[IBIS ver]   4.1
[File name]   sprm639a.ibs
[File Rev]   1.0
[Notes]
   IO cell model for C2000
[Date]   Nov 21, 2013
[Source]   File originated at Texas Instruments
[Copyright]   (c) 2012, Texas Instruments Inc.
[Component]   f771553xzwt
[Manufacturer] Texas Instruments
[Package]
| Variable   Typ   Min   Max
R_pkg   0.248   0.104   0.421
L_pkg   3.07E-09   9.51E-10   5.41E-09
C_pkg   7.15E-13   3.27E-13   1.18E-12
[Pin] signal_name   model_name   R_pin   L_pin   C_pin
A11   GPIO84   BCF3385DSHYPBFZ   0.319687   4.33705E-09   7.78071E-13
A12   GPIO153   BCF3350CSHYPBFZ   0.298822   4.20847E-09   6.39259E-13
A13   GPIO149   BCF3350CSHYPBFZ   0.342954   4.55481E-09   6.48797E-13
A14   GPIO81   BCF3385DSHYPBFZ   0.33134   4.4902E-09   7.50504E-13
A15   GPIO77   BCF3385DSHYPBFZ   0.337162   4.66581E-09   6.92522E-13
A16   GPIO73   BCF3385DSHYPBFZ   0.375286   4.90719E-09   9.3949E-13
A17   GPIO70   BCF3335DSHYPBFZ   0.421882   5.41022E-09   9.06764E-13
A2   GPIO97   BCF3385DSHYPBFZ   0.346517   3.88805E-09   7.27628E-13
A3   GPIO94   BCF3385DSHYPBFZ   0.327527   4.38519E-09   8.14171E-13
A4   GPIO92   BCF3385DSHYPBFZ   0.367132   4.84058E-09   8.98899E-13
A5   GPIO90   BCF3385DSHYPBFZ   0.309269   4.27709E-09   6.00141E-13
A6   GPIO6   GPIORETV2_NFS   0.308865   4.3618E-09   6.23916E-13
A7   GPIO2   GPIORETV2_NFS   0.295368   4.05632E-09   6.22769E-13
A8   GPIO163   BCF3350CSHYPBFZ   0.285759   3.62759E-09   7.23531E-13
|*A9,A18,B1,E7,E10,E13,F7,F10,F13,G5   VDDSFL   NC   0.146867   1.37666E-09   6.11163E-13*|
|*G6,H5,H6,L14,L15,M1,M5,M6,N14,N15,P9,R9,V19,W8   VDDSFL   NC   0.156081   1.50618E-09   6.11163E-13*|
B10   GPIO157   BCF3350CSHYPBFZ   0.309235   3.83913E-09   6.87623E-13
B11   GPIO85   BCF3385DSHYPBFZ   0.272894   3.41813E-09   7.01392E-13
B12   GPIO154   BCF3350CSHYPBFZ   0.303603   3.86334E-09   8.09406E-13
B13   GPIO150   BCF3350CSHYPBFZ   0.319404   4.36169E-09   8.51309E-13
B14   GPIO82   BCF3385DSHYPBFZ   0.287611   3.75595E-09   7.91276E-13
B15   GPIO78   BCF3385DSHYPBFZ   0.303045   3.86525E-09   9.89285E-13
B16   GPIO72   BCF3335DSHYPBFZ   0.320566   4.21723E-09   9.70252E-13
B17   GPIO71   BCF3385DSHYPBFZ   0.365339   4.78832E-09   8.84874E-13
B18   GPIO69   BCF3385DSHYPBFZ   0.377633   4.86821E-09   1.02379E-12
B19   GPIO67   BCF3385DSHYPBFZ   0.35161   3.71783E-09   9.11537E-13
B2   GPIO10   BCF183350CSHYPBFZ   0.304557   3.85412E-09   7.12492E-13
B3   GPIO95   BCF3350CSHYPBFZ   0.320186   4.02158E-09   7.8623E-13
B4   GPIO93   BCF3385DSHYPBFZ   0.320914   4.19498E-09   8.33886E-13
B5   GPIO91   BCF3385DSHYPBFZ   0.315637   4.16133E-09   9.379E-13
B6   GPIO7   GPIORETV2_NFS   0.252616   3.27964E-09   7.68154E-13
B7   GPIO3   GPIORETV2_NFS   0.248561   3.29545E-09   7.95932E-13
B8   GPIO164   BCF3350CSHYPBFZ   0.298994   3.61876E-09   6.752E-13
B9   GPIO160   BCF3350CSHYPBFZ   0.247443   3.09689E-09   5.80944E-13
C1   GPIO11   BCF183350CSHYPBFZ   0.307276   4.07789E-09   6.71632E-13
C10   GPIO158   BCF3350CSHYPBFZ   0.251923   3.02701E-09   6.50017E-13
C11   GPIO86   BCF3385DSHYPBFZ   0.240019   2.99169E-09   8.31328E-13
C12   GPIO155   BCF3350CSHYPBFZ   0.283764   3.59088E-09   7.34615E-13
C13   GPIO151   BCF3350CSHYPBFZ   0.25868   3.23014E-09   7.11853E-13
C14   GPIO83   BCF3385DSHYPBFZ   0.295575   3.78014E-09   7.76833E-13
C15   GPIO79   BCF3385DSHYPBFZ   0.31018   4.22638E-09   7.99064E-13
C16   GPIO76   BCF3385DSHYPBFZ   0.290281   3.78138E-09   1.02012E-12
C17   GPIO74   BCF3385DSHYPBFZ   0.323895   4.29426E-09   1.10069E-12
C18   GPIO68   BCF3385DSHYPBFZ   0.335665   3.64035E-09   1.10713E-12
C19   GPIO43   GPIOUSBV4_NFS_7LM   0.321464   3.65132E-09   7.88734E-13
C2   GPIO12   BCF183350CSHYPBFZ   0.292939   3.97645E-09   7.61513E-13
C3   GPIO96   BCF3385DSHYPBFZ   0.261803   3.07199E-09   8.01544E-13
C4   GPIO167   BCF3350CSHYPBFZ   0.294566   3.73299E-09   8.19332E-13
C5   GPIO165   BCF3350CSHYPBFZ   0.272342   3.43944E-09   6.65144E-13
C6   GPIO88   BCF3385DSHYPBFZ   0.259602   3.22338E-09   6.6121E-13
C7   GPIO4   GPIORETV2_NFS   0.215794   2.71638E-09   6.10609E-13
C8   GPIO0   GPIORETV2_NFS   0.244304   3.06821E-09   6.6699E-13
C9   GPIO161   BCF3350CSHYPBFZ   0.241226   2.87469E-09   7.86601E-13
D1   GPIO13   BCF183350CSHYPBFZ   0.299551   4.19571E-09   6.95654E-13
D10   GPIO159   BCF3350CSHYPBFZ   0.191658   2.18732E-09   7.58875E-13
D11   GPIO87   BCF3385DSHYPBFZ   0.22167   2.69751E-09   7.53613E-13
D12   GPIO156   BCF3350CSHYPBFZ   0.222483   2.73461E-09   8.74454E-13
D13   GPIO152   BCF3350CSHYPBFZ   0.248923   3.14502E-09   8.96352E-13
D14   GPIO148   BCF3350CSHYPBFZ   0.327228   4.26288E-09   9.56502E-13
D15   GPIO80   BCF3385DSHYPBFZ   0.325935   4.3086E-09   9.4736E-13
D16   GPIO75   BCF3385DSHYPBFZ   0.345154   4.59742E-09   9.19875E-13
D17   GPIO147   BCF3350CSHYPBFZ   0.26482   3.40869E-09   1.11582E-12
D18   GPIO146   BCF3350CSHYPBFZ   0.318138   3.82793E-09   1.18493E-12
D19   GPIO42   GPIOUSBV4_NFS_7LM   0.315732   4.00436E-09   7.19589E-13
D2   GPIO14   BCF183350CSHYPBFZ   0.307598   4.03173E-09   6.21597E-13
D3   GPIO15   BCF183350CSHYPBFZ   0.252167   3.22666E-09   7.94736E-13
D4   GPIO168   BCF3350CSHYPBFZ   0.226606   2.66721E-09   8.86402E-13
D5   GPIO166   BCF3350CSHYPBFZ   0.237854   3.0172E-09   7.4741E-13
D6   GPIO89   BCF3385DSHYPBFZ   0.206799   2.47062E-09   8.1398E-13
D7   GPIO5   GPIORETV2_NFS   0.192542   2.15668E-09   8.21398E-13
D8   GPIO1   GPIORETV2_NFS   0.168654   2.0599E-09   6.44669E-13
D9   GPIO162   BCF3350CSHYPBFZ   0.20821   2.27434E-09   5.90519E-13
E1   GPIO16   BCF183350CSHYPBFZ   0.314704   4.17604E-09   5.05103E-13
|*E16,F16   VDDSFL2   NC   0.156792   1.71059E-09   4.40263E-13*|
|*E16,F16   VDDSFL2   NC   0.154282   1.6878E-09   4.40263E-13*|
E17   GPIO145   BCF3350CSHYPBFZ   0.21249   2.55446E-09   9.60886E-13
E18   GPIO47   GPIOUSBV4_NFS_7LM   0.253816   3.03959E-09   6.70576E-13
E19   GPIO46   GPIOUSBV4_NFS_7LM   0.294305   3.60496E-09   6.48949E-13
E2   GPIO17   BCF183350CSHYPBFZ   0.257137   3.29303E-09   7.29543E-13
E3   GPIO18   BCF183350CSHYPBFZ   0.258589   3.34891E-09   5.60313E-13
E4   GPIO19   BCF183350CSHYPBFZ   0.27369   3.55971E-09   6.78789E-13
|*E9,E11,F9,F11,G14,G15,J14,J15,K5,K6,P10,P13,R10,R13   VDD   NC  0.171112   1.72645E-09   4.7223E-13*|
F1   GPIO98   BCF3385DSHYPBFZ   0.314572   4.25419E-09   6.22881E-13
F17   GPIO144   BCF3350BSHYPBFZ   0.237538   2.5957E-09   6.13332E-13
F18   GPIO143   BCF3350BSHYPBFZ   0.321464   4.16724E-09   1.01147E-12
F19   XRSn   BQ0491FS_3X2_7LM   0.286137   2.93417E-09   6.60717E-13
F2   GPIO20   BCF183350CSHYPBFZ   0.235787   3.13823E-09   6.44518E-13
F3   GPIO21   BCF183350CSHYPBFZ   0.244247   3.08261E-09   5.66615E-13
|*F4,G4   VDDSFL1833   NC   0.135167   1.53786E-09   5.04299E-13*|
|*F4,G4   VDDSFL1833   NC   0.126166   1.45446E-09   5.04299E-13*|
G1   GPIO99   BCF3385DSHYPBFZ   0.285592   3.81153E-09   7.64347E-13
G18   GPIO133   BCF3350BSHYPBFZ   0.294888   3.819E-09   7.35036E-13
G19   X1   NC   0.262328   2.90312E-09   7.47045E-13
G2   GPIO8   BCF3350CSHYPBFZ   0.264806   3.67528E-09   7.26003E-13
G3   GPIO9   BCF3350CSHYPBFZ   0.252788   3.25417E-09   6.09259E-13
H1   GPIO100   BCF3385DSHYPBFZ   0.263476   3.65228E-09   5.78824E-13
|*H16,H17   VDDSFL1   NC   0.133588   1.49772E-09   6.04206E-13*|
|*H16,H17   VDDSFL1   NC   0.13331   1.49845E-09   6.04206E-13*|
|*H18,H19   VSS   NC   0.232486   2.61579E-09   7.29732E-13*|
H2   GPIO101   BCF3385DSHYPBFZ   0.249794   3.18204E-09   5.27391E-13
H3   GPIO102   BCF3385DSHYPBFZ   0.226173   2.77789E-09   6.83769E-13
H4   VPP   NC   0.125134   1.44032E-09   3.27051E-13
J1   GPIO103   BCF3385DSHYPBFZ   0.287709   3.95912E-09   5.76491E-13
J16   GPIO63   BCF3385DSHYPBFZ   0.263216   2.95033E-09   8.91047E-13
J17   GPIO62   BCF3385DSHYPBFZ   0.30101   3.6262E-09   7.47986E-13
J18   VREGENZ   IQ0440FS_3X2_7LM   0.260757   3.23788E-09   6.52653E-13
J19   X2   NC   0.249184   3.17546E-09   6.96076E-13
J2   GPIO104   BCF3385DSHYPBFZ   0.223555   2.89779E-09   5.79891E-13
J3   GPIO105   BCF3385DSHYPBFZ   0.261577   3.22449E-09   6.38145E-13
J4   GPIO22   BCF3350CSHYPBFZ   0.211796   2.42294E-09   6.4932E-13
K1   GPIO26   BCF3350CSHYPBFZ   0.285128   3.9065E-09   6.35515E-13
K16   GPIO65   BCF3385DSHYPBFZ   0.174096   1.80345E-09   8.82989E-13
K17   GPIO66   BCF3335DSHYPBFZ   0.229966   2.57395E-09   5.41566E-13
K18   GPIO44   BCF3385DSHYPBFZ   0.271389   3.34545E-09   5.75478E-13
K19   GPIO45   BCF3385DSHYPBFZ   0.290096   4.03352E-09   6.51737E-13
K2   GPIO25   BCF3350CSHYPBFZ   0.234189   3.01207E-09   6.61863E-13
K3   GPIO24   BCF3350CSHYPBFZ   0.199766   2.32311E-09   5.45272E-13
K4   GPIO23   BCF3350CSHYPBFZ   0.142595   1.46053E-09   7.05502E-13
L1   GPIO27   BCF3350CSHYPBFZ   0.29442   3.97471E-09   6.61819E-13
L16   GPIO61   BCF3335DSHYPBFZ   0.133751   1.33372E-09   7.57122E-13
L17   GPIO64   BCF3335DSHYPBFZ   0.209578   2.25357E-09   5.83731E-13
L19   GPIO142   BCF3350BSHYPBFZ   0.306503   3.59516E-09   5.37682E-13
L2   GPIO106   BCF3385DSHYPBFZ   0.277201   3.4199E-09   5.17299E-13
L3   GPIO107   BCF3385DSHYPBFZ   0.220847   2.66337E-09   7.07224E-13
L4   GPIO108   BCF3385DSHYPBFZ   0.195261   2.03861E-09   5.37039E-13
M16   GPIO59   BCF3335DSHYPBFZ   0.134266   1.44911E-09   6.89352E-13
M17   GPIO60   BCF3385DSHYPBFZ   0.219583   2.23847E-09   8.61878E-13
M18   GPIO141   BCF3350BSHYPBFZ   0.287892   3.23826E-09   6.16719E-13
M19   GPIO140   BCF3350BSHYPBFZ   0.307057   3.82104E-09   6.32699E-13
M2   GPIO110   BCF3385DSHYPBFZ   0.283588   3.43407E-09   5.00861E-13
M3   GPIO112   BCF3385DSHYPBFZ   0.255848   2.93253E-09   5.7291E-13
M4   GPIO111   BCF3385DSHYPBFZ   0.179094   2.06636E-09   8.32478E-13
N16   GPIO56   BCF3385DSHYPBFZ   0.140094   1.67717E-09   7.26011E-13
N17   GPIO58   BCF3385DSHYPBFZ   0.239696   2.73931E-09   7.19111E-13
N18   GPIO57   BCF3385DSHYPBFZ   0.252681   3.14084E-09   5.55753E-13
N19   GPIO139   BCF3350BSHYPBFZ   0.32263   4.08555E-09   5.86096E-13
N2   GPIO109   BCF3385DSHYPBFZ   0.293848   3.66524E-09   7.64043E-13
N3   GPIO114   BCF3385DSHYPBFZ   0.273962   3.33937E-09   6.65314E-13
N4   GPIO113   BCF3385DSHYPBFZ   0.213519   2.56277E-09   7.61396E-13
|*P1,P5,R5,V7,W1   VSSA   NC   0.128935   1.30292E-09   9.97767E-13*|
|*P1,P5,R5,V7,W1   VSSA   NC   0.128558   1.41788E-09   9.97767E-13*|
|*P1,P5,R5,V7,W1   VSSA   NC   0.131821   1.42996E-09   9.97767E-13*|
|*P1,P5,R5,V7,W1   VSSA   NC   0.147367   1.47463E-09   9.97767E-13*|
|*P1,P5,R5,V7,W1   VSSA   NC   0.148848   1.45141E-09   9.97767E-13*|
|*P1,P5,R5,V7,W1   VSSA   NC   0.131419   1.3196E-09   9.97767E-13*|
P16   GPIO52   BCF3385DSHYPBFZ   0.24655   3.08807E-09   6.49119E-13
P17   GPIO53   BCF3385DSHYPBFZ   0.207708   2.86996E-09   5.95892E-13
P18   GPIO54   BCF3385DSHYPBFZ   0.263121   3.43701E-09   5.40139E-13
P19   GPIO55   BCF3385DSHYPBFZ   0.313207   4.21928E-09   6.49976E-13
P2   ADCINC1   NC   0.311442   4.01529E-09   6.9028E-13
P3   ADCINC3   NC   0.275666   3.47007E-09   7.11166E-13
P4   ADCINC5   NC   0.270084   3.25121E-09   9.143E-13
|*P6,R6   VDDA   NC   0.140595   1.46957E-09   4.04901E-13*|
|*P6,R6   VDDA   NC   0.143704   1.4855E-09   4.04901E-13*|
|*P6,R6   VDDA   NC   0.149119   1.6026E-09   4.04901E-13*|
|*P6,R6   VDDA   NC   0.14411   1.59172E-09   4.04901E-13*|
R1   VREFHI3   NC   0.292156   3.6476E-09   4.74414E-13
|*R11,R12   VDD3VFL   NC   0.117117   1.18661E-09   4.79636E-13*|
|*R11,R12   VDD3VFL   NC   0.115756   1.18172E-09   4.79636E-13*|
R16   GPIO48   BCF3385DSHYPBFZ   0.202473   2.42772E-09   6.9922E-13
R17   GPIO49   BCF3385DSHYPBFZ   0.211152   2.81544E-09   6.94346E-13
R18   GPIO50   BCF3385DSHYPBFZ   0.290055   3.84404E-09   6.44835E-13
R19   GPIO51   BCF3385DSHYPBFZ   0.313144   4.71586E-09   6.56413E-13
R2   ADCINC0   NC   0.318008   3.66132E-09   8.46127E-13
R3   ADCINC2   NC   0.279974   3.28028E-09   9.46719E-13
R4   ADCINC4   NC   0.305712   3.6984E-09   1.01504E-12
T1   ADCINA1   NC   0.379067   4.60718E-09   1.02321E-12
T10   GPIO129   BCF3350BSHYPBFZ   0.168143   2.075E-09   6.72018E-13
T11   GPIO30   BCF3355DSHYPBFZ   0.207085   2.45219E-09   8.10867E-13
T12   GPIO118   BCF3355DSHYPBFZ   0.187417   2.33318E-09   8.67819E-13
T13   GPIO33   BCF3385DSHYPBFZ   0.24449   2.84693E-09   7.57249E-13
T14   GPIO35   BCF3385DSHYPBFZ   0.279565   3.58098E-09   8.13795E-13
T15   GPIO119   BCF3385DSHYPBFZ   0.230666   2.73008E-09   7.94503E-13
T16   GPIO38   BCF3385DSHYPBFZ   0.236446   2.81408E-09   8.58047E-13
T17   GPIO136   BCF3350BSHYPBFZ   0.260209   3.18036E-09   7.40507E-13
T18   GPIO137   BCF3350BSHYPBFZ   0.253664   3.59979E-09   6.57827E-13
T19   GPIO138   BCF3350BSHYPBFZ   0.366548   5.03901E-09   7.07013E-13
T2   ADCINA3   NC   0.327198   4.02466E-09   9.03426E-13
T3   ADCINA5   NC   0.291696   3.43909E-09   8.41751E-13
T4   ADCINCAL0   NC   0.231734   2.60307E-09   7.77891E-13
T5   ADCIND0   NC   0.269236   3.20966E-09   1.0884E-12
T6   ADCIND2   NC   0.236315   2.66335E-09   9.76019E-13
T7   ADCIND4   NC   0.201937   2.21871E-09   8.76865E-13
T8   GPIO122   BCF3350CSHYPBFZ   0.188754   2.03765E-09   7.57926E-13
T9   GPIO125   BCF3350CSHYPBFZ   0.192836   2.24227E-09   5.7875E-13
U1   ADCINA0   NC   0.37235   4.01208E-09   9.42551E-13
U10   GPIO130   BCF3350BSHYPBFZ   0.234168   2.75572E-09   7.21435E-13
U11   GPIO31   BCF3385DSHYPBFZ   0.23223   2.89131E-09   8.5392E-13
U12   GPIO117   BCF3385DSHYPBFZ   0.254774   3.22477E-09   7.05375E-13
U13   GPIO32   BCF3385DSHYPBFZ   0.251017   3.07874E-09   8.00807E-13
U14   GPIO34   BCF3385DSHYPBFZ   0.292993   3.92802E-09   8.95378E-13
U15   GPIO120   BCF3385DSHYPBFZ   0.262186   3.28134E-09   8.302E-13
U16   GPIO37   BCF3385DSHYPBFZ   0.299968   3.81805E-09   7.77713E-13
U17   GPIO41   BCF3385DSHYPBFZ   0.267542   3.19136E-09   7.89233E-13
U18   GPIO135   BCF3350BSHYPBFZ   0.282532   3.57465E-09   8.07922E-13
U19   ERRORSTS   BCF3350BSHYPBFZ   0.331871   4.97925E-09   7.70725E-13
U2   ADCINA2   NC   0.311298   3.71659E-09   8.8044E-13
U3   ADCINA4   NC   0.318402   3.83269E-09   9.60795E-13
U4   ADCINCAL1   NC   0.228454   2.67067E-09   7.52549E-13
U5   ADCIND1   NC   0.326764   4.05111E-09   9.9439E-13
U6   ADCIND3   NC   0.290201   3.53878E-09   8.82E-13
U7   ADCIND5   NC   0.253388   3.03004E-09   6.81758E-13
U8   GPIO123   BCF3350CSHYPBFZ   0.242641   3.11525E-09   6.3312E-13
U9   GPIO126   BCF3350BSHYPBFZ   0.185925   2.22287E-09   6.93075E-13
V1   VREFHI1   NC   0.369535   5.40512E-09   5.30551E-13
V10   GPIO131   BCF3350BSHYPBFZ   0.279504   3.37507E-09   6.6615E-13
V11   GPIO28   BCF3385DSHYPBFZ   0.255649   3.28444E-09   8.29621E-13
V12   GPIO115   BCF3385DSHYPBFZ   0.288069   3.65968E-09   7.14266E-13
V13   FLT2   NC   0.305298   4.10153E-09   8.58332E-13
V14   TRSTn   BCF3335CSHYPBFZ   0.283791   3.63946E-09   6.4083E-13
V15   TCK   IQ0442FS_40P60P_3X2   0.286895   3.78615E-09   6.4391E-13
V16   GPIO36   BCF3385DSHYPBFZ   0.313618   3.97607E-09   7.58104E-13
V17   GPIO40   BCF3385DSHYPBFZ   0.323102   3.69501E-09   8.09236E-13
V18   GPIO134   BCF3350BSHYPBFZ   0.309784   3.42121E-09   7.53338E-13
V2   ADCINB0   NC   0.337471   4.33747E-09   9.8716E-13
V3   ADCINB2   NC   0.314177   4.12581E-09   9.0581E-13
V4   ADCINB4   NC   0.281766   3.6898E-09   8.24867E-13
V5   VREFHI4   NC   0.296639   3.85095E-09   5.72503E-13
V6   ADCINB6   NC   0.267778   3.38078E-09   9.40434E-13
V8   GPIO124   BCF3350CSHYPBFZ   0.27037   2.97807E-09   7.1671E-13
V9   GPIO127   BCF3350BSHYPBFZ   0.243386   3.23487E-09   5.7448E-13
W10   GPIO116   BCF3385DSHYPBFZ   0.323301   4.29268E-09   7.24081E-13
W11   GPIO29   BCF3385DSHYPBFZ   0.312781   4.07535E-09   6.64261E-13
W12   FLT1   NC   0.365722   5.03529E-09   7.40279E-13
W13   TDI   BCF3335DSHYPBFZ   0.347649   4.82237E-09   6.78258E-13
W14   TMS   IQ0442FS_40P60P_3X2   0.316961   4.44717E-09   6.37992E-13
W15   TDO   BCF3335DSHYPBFZ   0.306073   4.36739E-09   7.01858E-13
W16   GPIO121   BCF3385DSHYPBFZ   0.343232   4.66495E-09   6.67902E-13
W17   GPIO39   BCF3385DSHYPBFZ   0.34051   4.20726E-09   7.38362E-13
W18   GPIO132   BCF3350BSHYPBFZ   0.350769   4.46255E-09   8.43315E-13
W2   ADCINB1   NC   0.366887   5.03667E-09   9.55694E-13
W3   ADCINB3   NC   0.331552   4.5358E-09   8.71018E-13
W4   ADCINB5   NC   0.323419   4.30425E-09   7.87175E-13
W5   VREFHI2   NC   0.301864   4.10299E-09   4.93885E-13
W6   ADCINB7   NC   0.311213   4.08957E-09   9.5351E-13
W9   GPIO128   BCF3350BSHYPBFZ   0.27912   3.76947E-09   6.2859E-13
| End of package information
|   Component BCF3335DSHYPBFZ
[Component]   BCF3335DSHYPBFZ
[Manufacturer]   Texas Instruments
[Package]
|  variable   typ   min   max
R_pkg   0   0   0
L_pkg   0   0   0
C_pkg   0   0   0
[Pin]   signal_name   model_name   R_pin   L_pin   C_pin
VSS   VSS   GND
VDDS   VDDS   POWER
PAD   PAD   BCF3335DSHYPBFZ
[Model Selector] BCF3335DSHYPBFZ
BCF3335D_WK_PU_ON  Cell operated at 3.3(nom)
|BCF3335D_WK_PU_ON; WEAK_PULLUP_ON
BCF3335D_DRIVER_MODE  Cell operated at 3.3(nom)
|BCF3335D_DRIVER_MODE
BCF3335D_WK_PD_ON  Cell operated at 3.3(nom)
|   Component BCF3385DSHYPBFZ
[Component]   BCF3385DSHYPBFZ
[Manufacturer]   Texas Instruments
[Package]
|  variable   typ   min   max
R_pkg   0   0   0
L_pkg   0   0   0
C_pkg   0   0   0
[Pin]   signal_name   model_name   R_pin   L_pin   C_pin
VSS   VSS   GND
VDDS   VDDS   POWER
PAD   PAD   BCF3385DSHYPBFZ
[Model Selector] BCF3385DSHYPBFZ
BCF3385D_WK_PU_ON  Cell operated at 3.3(nom)
|BCF3385D_WK_PU_ON; WEAK_PULLUP_ON
BCF3385D_DRIVER_MODE  Cell operated at 3.3(nom)
|BCF3385D_DRIVER_MODE
BCF3385D_WK_PD_ON  Cell operated at 3.3(nom)
|   Component BCF183350CSHYPBFZ
[Component]   BCF183350CSHYPBFZ
[Manufacturer]   Texas Instruments
[Package]
|  variable   typ   min   max
R_pkg   0   0   0
L_pkg   0   0   0
C_pkg   0   0   0
[Pin]   signal_name   model_name   R_pin   L_pin   C_pin
VSS   VSS   GND
VDDS   VDDS   POWER
PAD   PAD   BCF183350CSHYPBFZ
[Model Selector] BCF183350CSHYPBFZ
BCF183350C_WK_PU_ON_3P3V  Cell operated at 3.3(nom)
|BCF183350C_WK_PU_ON_3P3V; WEAK_PULLUP_ON
BCF183350C_DRVR_MODE_3P3V  Cell operated at 3.3(nom)
|BCF183350C_DRVR_MODE_3P3V
BCF183350C_WK_PD_ON_3P3V  Cell operated at 3.3(nom)
|BCF183350C_WK_PD_ON_3P3V; WEAK_PULLDOWN_ON
BCF183350C_WK_PU_ON_1P8  Cell operated at 1.8(nom)
|BCF183350C_WK_PU_ON_1P8; WEAK_PULLUP_ON
BCF183350C_DRVR_MODE_1P8  Cell operated at 1.8(nom)
|BCF183350C_DRVR_MODE_1P8
BCF183350C_WK_PD_ON_1P8  Cell operated at 1.8(nom)
|   Component IQ0442FS_40P60P_3X2
[Component]   IQ0442FS_40P60P_3X2
[Manufacturer]   Texas Instruments
[Package]
|  variable   typ   min   max
R_pkg   0   0   0
L_pkg   0   0   0
C_pkg   0   0   0
[Pin]   signal_name   model_name   R_pin   L_pin   C_pin
VSS   VSS   GND
VDDS   VDDS   POWER
PAD   PAD   IQ0442FS_40P60P_3X2
[Model Selector] IQ0442FS_40P60P_3X2
S_40P60P_3X2_7LM_3P3  Cell operated at 3.3(nom)
|IQ0442FS_40P60P_3X2_3P3; PUPD_OFF
0P60P_3X2_7LM_PU_3P3  Cell operated at 3.3(nom)
|IQ0442FS_40P60P_3X2_PU_3P3; PULLUP_ON
0P60P_3X2_7LM_PD_3P3  Cell operated at 3.3(nom)
|   Component IQ0440FS_3X2_7LM
[Component]   IQ0440FS_3X2_7LM
[Manufacturer]   Texas Instruments
[Package]
|  variable   typ   min   max
R_pkg   0   0   0
L_pkg   0   0   0
C_pkg   0   0   0
[Pin]   signal_name   model_name   R_pin   L_pin   C_pin
VSS   VSS   GND
VDDS   VDDS   POWER
PAD   PAD   IQ0440FS_3X2_7LM
[Model Selector] IQ0440FS_3X2_7LM
440FS_3X2_7LM_PD_3P3  Cell operated at 3.3(nom)
|IQ0440FS_3X2_7LM_PD_3P3; PULLDOWN_ON
IQ0440FS_3X2_7LM_3P3  Cell operated at 3.3(nom)
|   Component BQ0491FS_3X2_7LM
[Component]   BQ0491FS_3X2_7LM
[Manufacturer]   Texas Instruments
[Package]
|  variable   typ   min   max
R_pkg   0   0   0
L_pkg   0   0   0
C_pkg   0   0   0
[Pin]   signal_name   model_name   R_pin   L_pin   C_pin
VSS   VSS   GND
VDDS   VDDS   POWER
PAD   PAD   BQ0491FS_3X2_7LM
[Model Selector] BQ0491FS_3X2_7LM
491FS_3X2_7LM_PU_3P3  Cell operated at 3.3(nom)
|BQ0491FS_3X2_7LM_PU_3P3; PULLUP_ON
491FS_3X2_7LM_PZ_3P3  Cell operated at 3.3(nom)
|   Component GPIORETV2_NFS
[Component]   GPIORETV2_NFS
[Manufacturer]   Texas Instruments
[Package]
|  variable   typ   min   max
R_pkg   0   0   0
L_pkg   0   0   0
C_pkg   0   0   0
[Pin]   signal_name   model_name   R_pin   L_pin   C_pin
VSS   VSS   GND
VDDS   VDDS   POWER
PAD   PAD   GPIORETV2_NFS
[Model Selector] GPIORETV2_NFS
GPIORET_WK_PD_ON_3P3  Cell operated at 3.3(nom)
|GPIORET_WK_PD_ON_3P3; WEAK_PULLDOWN_ON
RET_8MA_OPEN_DRAIN  Cell operated at 3.3(nom)
|RET_8MA_OPEN_DRAIN; 8MA_OPEN_DRAIN_SLW
RET_DRVR_2MA_PUPDOFF  Cell operated at 3.3(nom)
|RET_DRVR_2MA_PUPDOFF
RET_4MA_OPEN_DRAIN  Cell operated at 3.3(nom)
|RET_4MA_OPEN_DRAIN; 4MA_OPEN_DRAIN
GPIORET_WK_PU_ON_3P3  Cell operated at 3.3(nom)
|GPIORET_WK_PU_ON_3P3; WEAK_PULLUP_ON
RET_2MA_OPEN_DRAIN  Cell operated at 3.3(nom)
|RET_2MA_OPEN_DRAIN; 2MA_OPEN_DRAIN
RET_DRVR_8MA_PUPDOFF  Cell operated at 3.3(nom)
|RET_DRVR_8MA_PUPDOFF
RET_DRVR_MODE_8MA_PUPDOFF_SLEW  Cell operated at 3.3(nom)
|RET_DRVR_MODE_8MA_PUPDOFF_SLEW
RET_DRVR_MODE_4MA_PUPDOFF  Cell operated at 3.3(nom)
|RET_DRVR_MODE_4MA_PUPDOFF
RET_8MA_OPEN_DRAIN_3P3  Cell operated at 3.3(nom)
|   Component BCF3335CSHYPBFZ
[Component]   BCF3335CSHYPBFZ
[Manufacturer]   Texas Instruments
[Package]
|  variable   typ   min   max
R_pkg   0   0   0
L_pkg   0   0   0
C_pkg   0   0   0
[Pin]   signal_name   model_name   R_pin   L_pin   C_pin
VSS   VSS   GND
VDDS   VDDS   POWER
PAD   PAD   BCF3335CSHYPBFZ
[Model Selector] BCF3335CSHYPBFZ
BCF3335C_WK_PU_ON_3P3  Cell operated at 3.3(nom)
|BCF3335C_WK_PU_ON_3P3; WEAK_PULLUP_ON
BCF3335C_DRIVER_MODE_3P3  Cell operated at 3.3(nom)
|BCF3335C_DRIVER_MODE_3P3
BCF3335C_WK_PD_ON_3P3  Cell operated at 3.3(nom)
|   Component BCF3350CSHYPBFZ
[Component]   BCF3350CSHYPBFZ
[Manufacturer]   Texas Instruments
[Package]
|  variable   typ   min   max
R_pkg   0   0   0
L_pkg   0   0   0
C_pkg   0   0   0
[Pin]   signal_name   model_name   R_pin   L_pin   C_pin
VSS   VSS   GND
VDDS   VDDS   POWER
PAD   PAD   BCF3350CSHYPBFZ
[Model Selector] BCF3350CSHYPBFZ
BCF3350C_WK_PU_ON_3P3  Cell operated at 3.3(nom)
|BCF3350C_WK_PU_ON_3P3; WEAK_PULLUP_ON
BCF3350C_DRIVER_MODE_3P3  Cell operated at 3.3(nom)
|BCF3350C_DRIVER_MODE_3P3
BCF3350C_WK_PD_ON_3P3  Cell operated at 3.3(nom)
|   Component BCF3350BSHYPBFZ
[Component]   BCF3350BSHYPBFZ
[Manufacturer]   Texas Instruments
[Package]
|  variable   typ   min   max
R_pkg   0   0   0
L_pkg   0   0   0
C_pkg   0   0   0
[Pin]   signal_name   model_name   R_pin   L_pin   C_pin
VSS   VSS   GND
VDDS   VDDS   POWER
PAD   PAD   BCF3350BSHYPBFZ
[Model Selector] BCF3350BSHYPBFZ
BCF3350B_WK_PU_ON_3P3  Cell operated at 3.3(nom)
|BCF3350B_WK_PU_ON_3P3; WEAK_PULLUP_ON
BCF3350B_DRIVER_MODE_3P3  Cell operated at 3.3(nom)
|BCF3350B_DRIVER_MODE_3P3
BCF3350B_WK_PD_ON_3P3  Cell operated at 3.3(nom)
|   Component GPIOUSBV4_NFS_7LM
[Component]   GPIOUSBV4_NFS_7LM
[Manufacturer]   Texas Instruments
[Package]
|  variable   typ   min   max
R_pkg   0   0   0
L_pkg   0   0   0
C_pkg   0   0   0
[Pin]   signal_name   model_name   R_pin   L_pin   C_pin
VSS   VSS   GND
VDDS   VDDS   POWER
PAD   PAD   GPIOUSBV4_NFS_7LM
[Model Selector] GPIOUSBV4_NFS_7LM
GPIOUSB_WK_PD_ON_3P3  Cell operated at 3.3(nom)
|GPIOUSB_WK_PD_ON_3P3; WEAK_PULLDOWN_ON
USB_8MA_OPEN_DRAIN_SLW  Cell operated at 3.3(nom)
|USB_8MA_OPEN_DRAIN_SLW; 8MA_OPEN_DRAIN_SLW
USB_DRVR_2MA_PUPDOFF  Cell operated at 3.3(nom)
|USB_DRVR_2MA_PUPDOFF
USB_4MA_OPEN_DRAIN  Cell operated at 3.3(nom)
|USB_4MA_OPEN_DRAIN; 4MA_OPEN_DRAIN
GPIOUSB_WK_PU_ON_3P3  Cell operated at 3.3(nom)
|GPIOUSB_WK_PU_ON_3P3; WEAK_PULLUP_ON
USB_2MA_OPEN_DRAIN  Cell operated at 3.3(nom)
|USB_2MA_OPEN_DRAIN; 2MA_OPEN_DRAIN
USB_DRVR_8MA_PUPDOFF  Cell operated at 3.3(nom)
|USB_DRVR_8MA_PUPDOFF
USB_DRVR_8MA_PUPDOFF_SLW  Cell operated at 3.3(nom)
|USB_DRVR_8MA_PUPDOFF_SLW
USB_DRVR_4MA_PUPDOFF  Cell operated at 3.3(nom)
|USB_DRVR_4MA_PUPDOFF
USB_8MA_OPEN_DRAIN  Cell operated at 3.3(nom)
|   Component BCF3355DSHYPBFZ
[Component]   BCF3355DSHYPBFZ
[Manufacturer]   Texas Instruments
[Package]
|  variable   typ   min   max
R_pkg   0   0   0
L_pkg   0   0   0
C_pkg   0   0   0
[Pin]   signal_name   model_name   R_pin   L_pin   C_pin
VSS   VSS   GND
VDDS   VDDS   POWER
PAD   PAD   BCF3355DSHYPBFZ
[Model Selector] BCF3355DSHYPBFZ
BCF3355D_WK_PU_ON_3P3  Cell operated at 3.3(nom)
|BCF3355D_WK_PU_ON_3P3; WEAK_PULLUP_ON
BCF3355D_DRIVER_MODE_3P3  Cell operated at 3.3(nom)
|BCF3355D_DRIVER_MODE_3P3
BCF3355D_WK_PD_ON_3P3  Cell operated at 3.3(nom)
| Models and submodels in the file (51): BCF3335D_WK_PU_ON (Input), BCF3335D_DRIVER_MODE (I/O), BCF3335D_WK_PD_ON (Input), BCF3385D_WK_PU_ON (Input), BCF3385D_DRIVER_MODE (I/O), BCF3385D_WK_PD_ON (Input), BCF183350C_WK_PU_ON_1P8 (Input), BCF183350C_DRVR_MODE_1P8 (I/O), BCF183350C_WK_PD_ON_1P8 (Input), BCF183350C_WK_PU_ON_3P3V (Input), BCF183350C_DRVR_MODE_3P3V (I/O), BCF183350C_WK_PD_ON_3P3V (Input), S_40P60P_3X2_7LM_3P3 (Input), 0P60P_3X2_7LM_PU_3P3 (Input), 0P60P_3X2_7LM_PD_3P3 (Input), 440FS_3X2_7LM_PD_3P3 (Input), IQ0440FS_3X2_7LM_3P3 (Input), 491FS_3X2_7LM_PU_3P3 (I/O), 491FS_3X2_7LM_PZ_3P3 (I/O), GPIORET_WK_PD_ON_3P3 (Input), RET_8MA_OPEN_DRAIN (I/O_open_drain), RET_DRVR_2MA_PUPDOFF (I/O), RET_4MA_OPEN_DRAIN (I/O_open_drain), GPIORET_WK_PU_ON_3P3 (Input), RET_2MA_OPEN_DRAIN (I/O_open_drain), RET_DRVR_8MA_PUPDOFF (I/O), RET_DRVR_MODE_8MA_PUPDOFF_SLEW (I/O), RET_DRVR_MODE_4MA_PUPDOFF (I/O), RET_8MA_OPEN_DRAIN_3P3 (I/O_open_drain), BCF3335C_WK_PU_ON_3P3 (Input), BCF3335C_DRIVER_MODE_3P3 (I/O), BCF3335C_WK_PD_ON_3P3 (Input), BCF3350C_WK_PU_ON_3P3 (Input), BCF3350C_DRIVER_MODE_3P3 (I/O), BCF3350C_WK_PD_ON_3P3 (Input), BCF3350B_WK_PU_ON_3P3 (Input), BCF3350B_DRIVER_MODE_3P3 (I/O), BCF3350B_WK_PD_ON_3P3 (Input), GPIOUSB_WK_PD_ON_3P3 (Input), USB_8MA_OPEN_DRAIN_SLW (I/O_open_drain), USB_DRVR_2MA_PUPDOFF (I/O), USB_4MA_OPEN_DRAIN (I/O_open_drain), GPIOUSB_WK_PU_ON_3P3 (Input), USB_2MA_OPEN_DRAIN (I/O_open_drain), USB_DRVR_8MA_PUPDOFF (I/O), USB_DRVR_8MA_PUPDOFF_SLW (I/O), USB_DRVR_4MA_PUPDOFF (I/O), USB_8MA_OPEN_DRAIN (I/O_open_drain), BCF3355D_WK_PU_ON_3P3 (Input), BCF3355D_DRIVER_MODE_3P3 (I/O), BCF3355D_WK_PD_ON_3P3 (Input)
